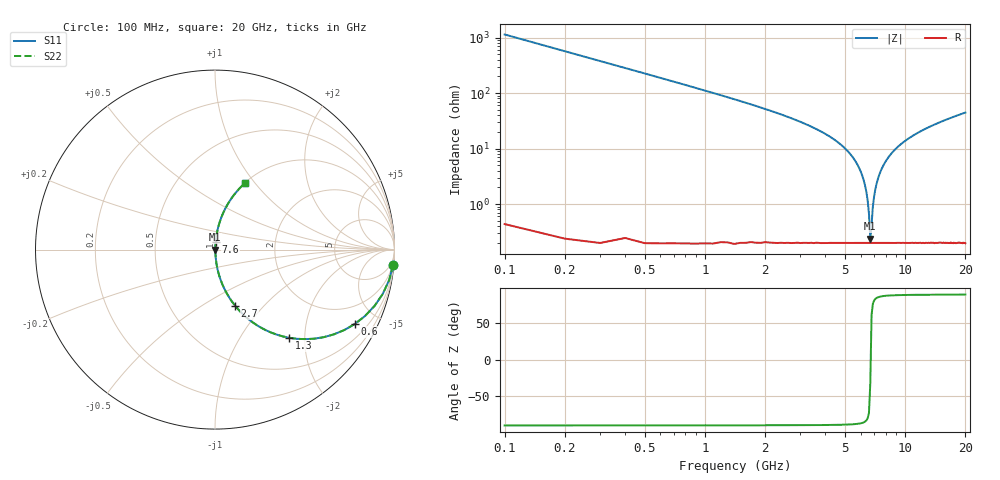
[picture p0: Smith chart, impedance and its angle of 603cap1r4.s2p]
! AVX Thin Film Operation		Date: November 2004
! Description: Accu-P® Series, Thin Film, SMD, RF Capacitor
! Part Number: 06035J1R4ABT
! 50 MHz  -  10.05 GHz
! Serial Measurements
# hz S db R 50
!	S11		S21		S12		S22
!	dB	Phase	dB	Phase	dB	Phase	dB	Phase
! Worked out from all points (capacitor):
!   200 points, 100 MHz to 20 GHz, reference 50 ohm
!   read as one part in series: C = 1.4 pF near 200 MHz
!   lowest |Z| = 238 mohm at 6.7 GHz (marker M1)
!   series resonance near 6.726 GHz, so ESL is about 400 pH
!   S11 on the Smith chart (normalised r, x): 100 MHz: 1, -23; 600 MHz: 1.00, -3.76; 1.3 GHz: 1.00, -1.68; 2.7 GHz: 1.00, -0.71; 7.6 GHz: 1.00, +0.08; 20 GHz: 1.00, +0.89
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1e8  -0.03 -5.0  -21.15 85.0  -21.15 85.0  -0.03 -5.0
2e8  -0.13 -10.0  -15.22 80.0  -15.22 80.0  -0.13 -10.0
3e8  -0.29 -14.8  -11.85 75.2  -11.85 75.2  -0.29 -14.8
6e8  -1.09 -28.0  -6.57 61.9  -6.57 61.9  -1.09 -28.0
1.3e9  -3.83 -49.8  -2.34 40.0  -2.34 40.0  -3.83 -49.8
2.7e9  -9.57 -70.3  -0.53 19.4  -0.53 19.4  -9.57 -70.3
3.5e9  -12.76 -76.2  -0.25 13.3  -0.25 13.3  -12.76 -76.2
5.1e9  -20.52 -83.4  -0.06 5.4  -0.06 5.4  -20.52 -83.4
6e9  -28.26 -84.8  -0.02 2.2  -0.02 2.2  -28.26 -84.8
6.3e9  -33.09 -83.6  -0.02 1.3  -0.02 1.3  -33.09 -83.6
6.5e9  -38.65 -79.5  -0.02 0.7  -0.02 0.7  -38.65 -79.5
6.6e9  -43.53 -72.2  -0.02 0.4  -0.02 0.4  -43.53 -72.2
6.7e9  -52.49 -32.6  -0.02 0.1  -0.02 0.1  -52.49 -32.6
6.8e9  -47.50 61.5  -0.02 -0.2  -0.02 -0.2  -47.50 61.5
6.9e9  -41.04 76.5  -0.02 -0.5  -0.02 -0.5  -41.04 76.5
7.1e9  -34.71 82.7  -0.02 -1.0  -0.02 -1.0  -34.71 82.7
7.6e9  -27.67 84.9  -0.02 -2.4  -0.02 -2.4  -27.67 84.9
8.6e9  -21.56 83.8  -0.05 -4.8  -0.05 -4.8  -21.56 83.8
1.01e10  -17.10 81.2  -0.10 -8.0  -0.10 -8.0  -17.10 81.2
1.34e10  -12.26 75.4  -0.28 -14.1  -0.28 -14.1  -12.26 75.4
1.67e10  -9.60 70.3  -0.52 -19.3  -0.52 -19.3  -9.60 70.3
2e10  -7.82 65.8  -0.80 -24.0  -0.80 -24.0  -7.82 65.8
